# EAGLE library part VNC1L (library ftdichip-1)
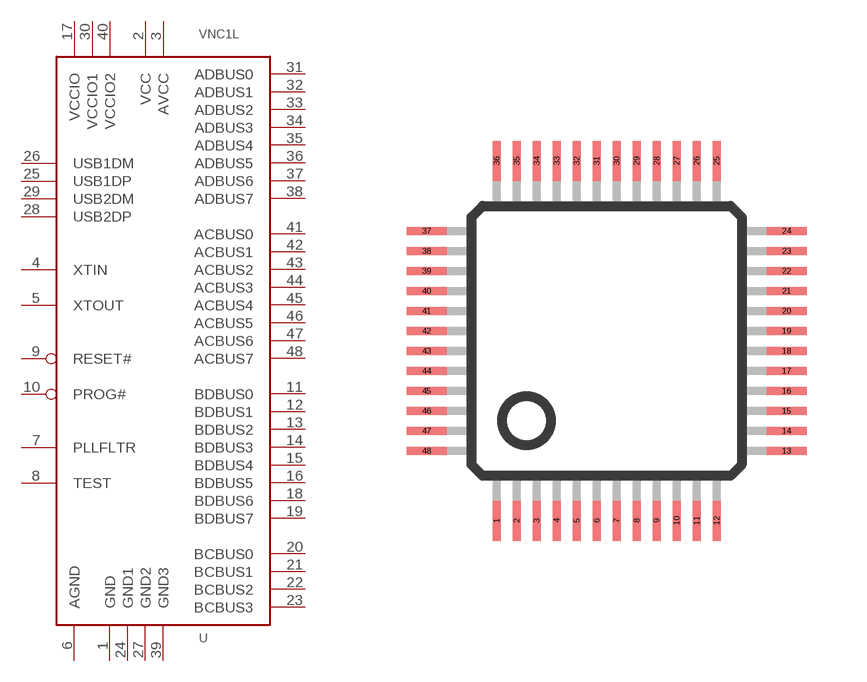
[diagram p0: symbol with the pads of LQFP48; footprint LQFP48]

Designator prefix U

## VNC1L-1A  [LQFP48]
1  GND  pwr
2  VCC  pwr
3  AVCC  pwr
4  XTIN  in
5  XTOUT  out
6  AGND  pwr
7  PLLFLTR  in
8  TEST  in
9  RESET#  in
10  PROG#  in
11  BDBUS0
12  BDBUS1
13  BDBUS2
14  BDBUS3
15  BDBUS4
16  BDBUS5
17  VCCIO  pwr
18  BDBUS6
19  BDBUS7
20  BCBUS0
21  BCBUS1
22  BCBUS2
23  BCBUS3
24  GND1  pwr
25  USB1DP
26  USB1DM
27  GND2  pwr
28  USB2DP
29  USB2DM
30  VCCIO1  pwr
31  ADBUS0
32  ADBUS1
33  ADBUS2
34  ADBUS3
35  ADBUS4
36  ADBUS5
37  ADBUS6
38  ADBUS7
39  GND3  pwr
40  VCCIO2  pwr
41  ACBUS0
42  ACBUS1
43  ACBUS2
44  ACBUS3
45  ACBUS4
46  ACBUS5
47  ACBUS6
48  ACBUS7

## Footprint LQFP48 (pad centres in mm)
smd 0.2 x 1: 1 -2.75,-4.5; 2 -2.25,-4.5; 3 -1.75,-4.5; 4 -1.25,-4.5; 5 -0.75,-4.5; 6 -0.25,-4.5; 7 0.25,-4.5; 8 0.75,-4.5; 9 1.25,-4.5; 10 1.75,-4.5; 11 2.25,-4.5; 12 2.75,-4.5; 25 2.75,4.5; 26 2.25,4.5; 27 1.75,4.5; 28 1.25,4.5; 29 0.75,4.5; 30 0.25,4.5; 31 -0.25,4.5; 32 -0.75,4.5; 33 -1.25,4.5; 34 -1.75,4.5; 35 -2.25,4.5; 36 -2.75,4.5
smd 1 x 0.2: 13 4.5,-2.75; 14 4.5,-2.25; 15 4.5,-1.75; 16 4.5,-1.25; 17 4.5,-0.75; 18 4.5,-0.25; 19 4.5,0.25; 20 4.5,0.75; 21 4.5,1.25; 22 4.5,1.75; 23 4.5,2.25; 24 4.5,2.75; 37 -4.5,2.75; 38 -4.5,2.25; 39 -4.5,1.75; 40 -4.5,1.25; 41 -4.5,0.75; 42 -4.5,0.25; 43 -4.5,-0.25; 44 -4.5,-0.75; 45 -4.5,-1.25; 46 -4.5,-1.75; 47 -4.5,-2.25; 48 -4.5,-2.75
